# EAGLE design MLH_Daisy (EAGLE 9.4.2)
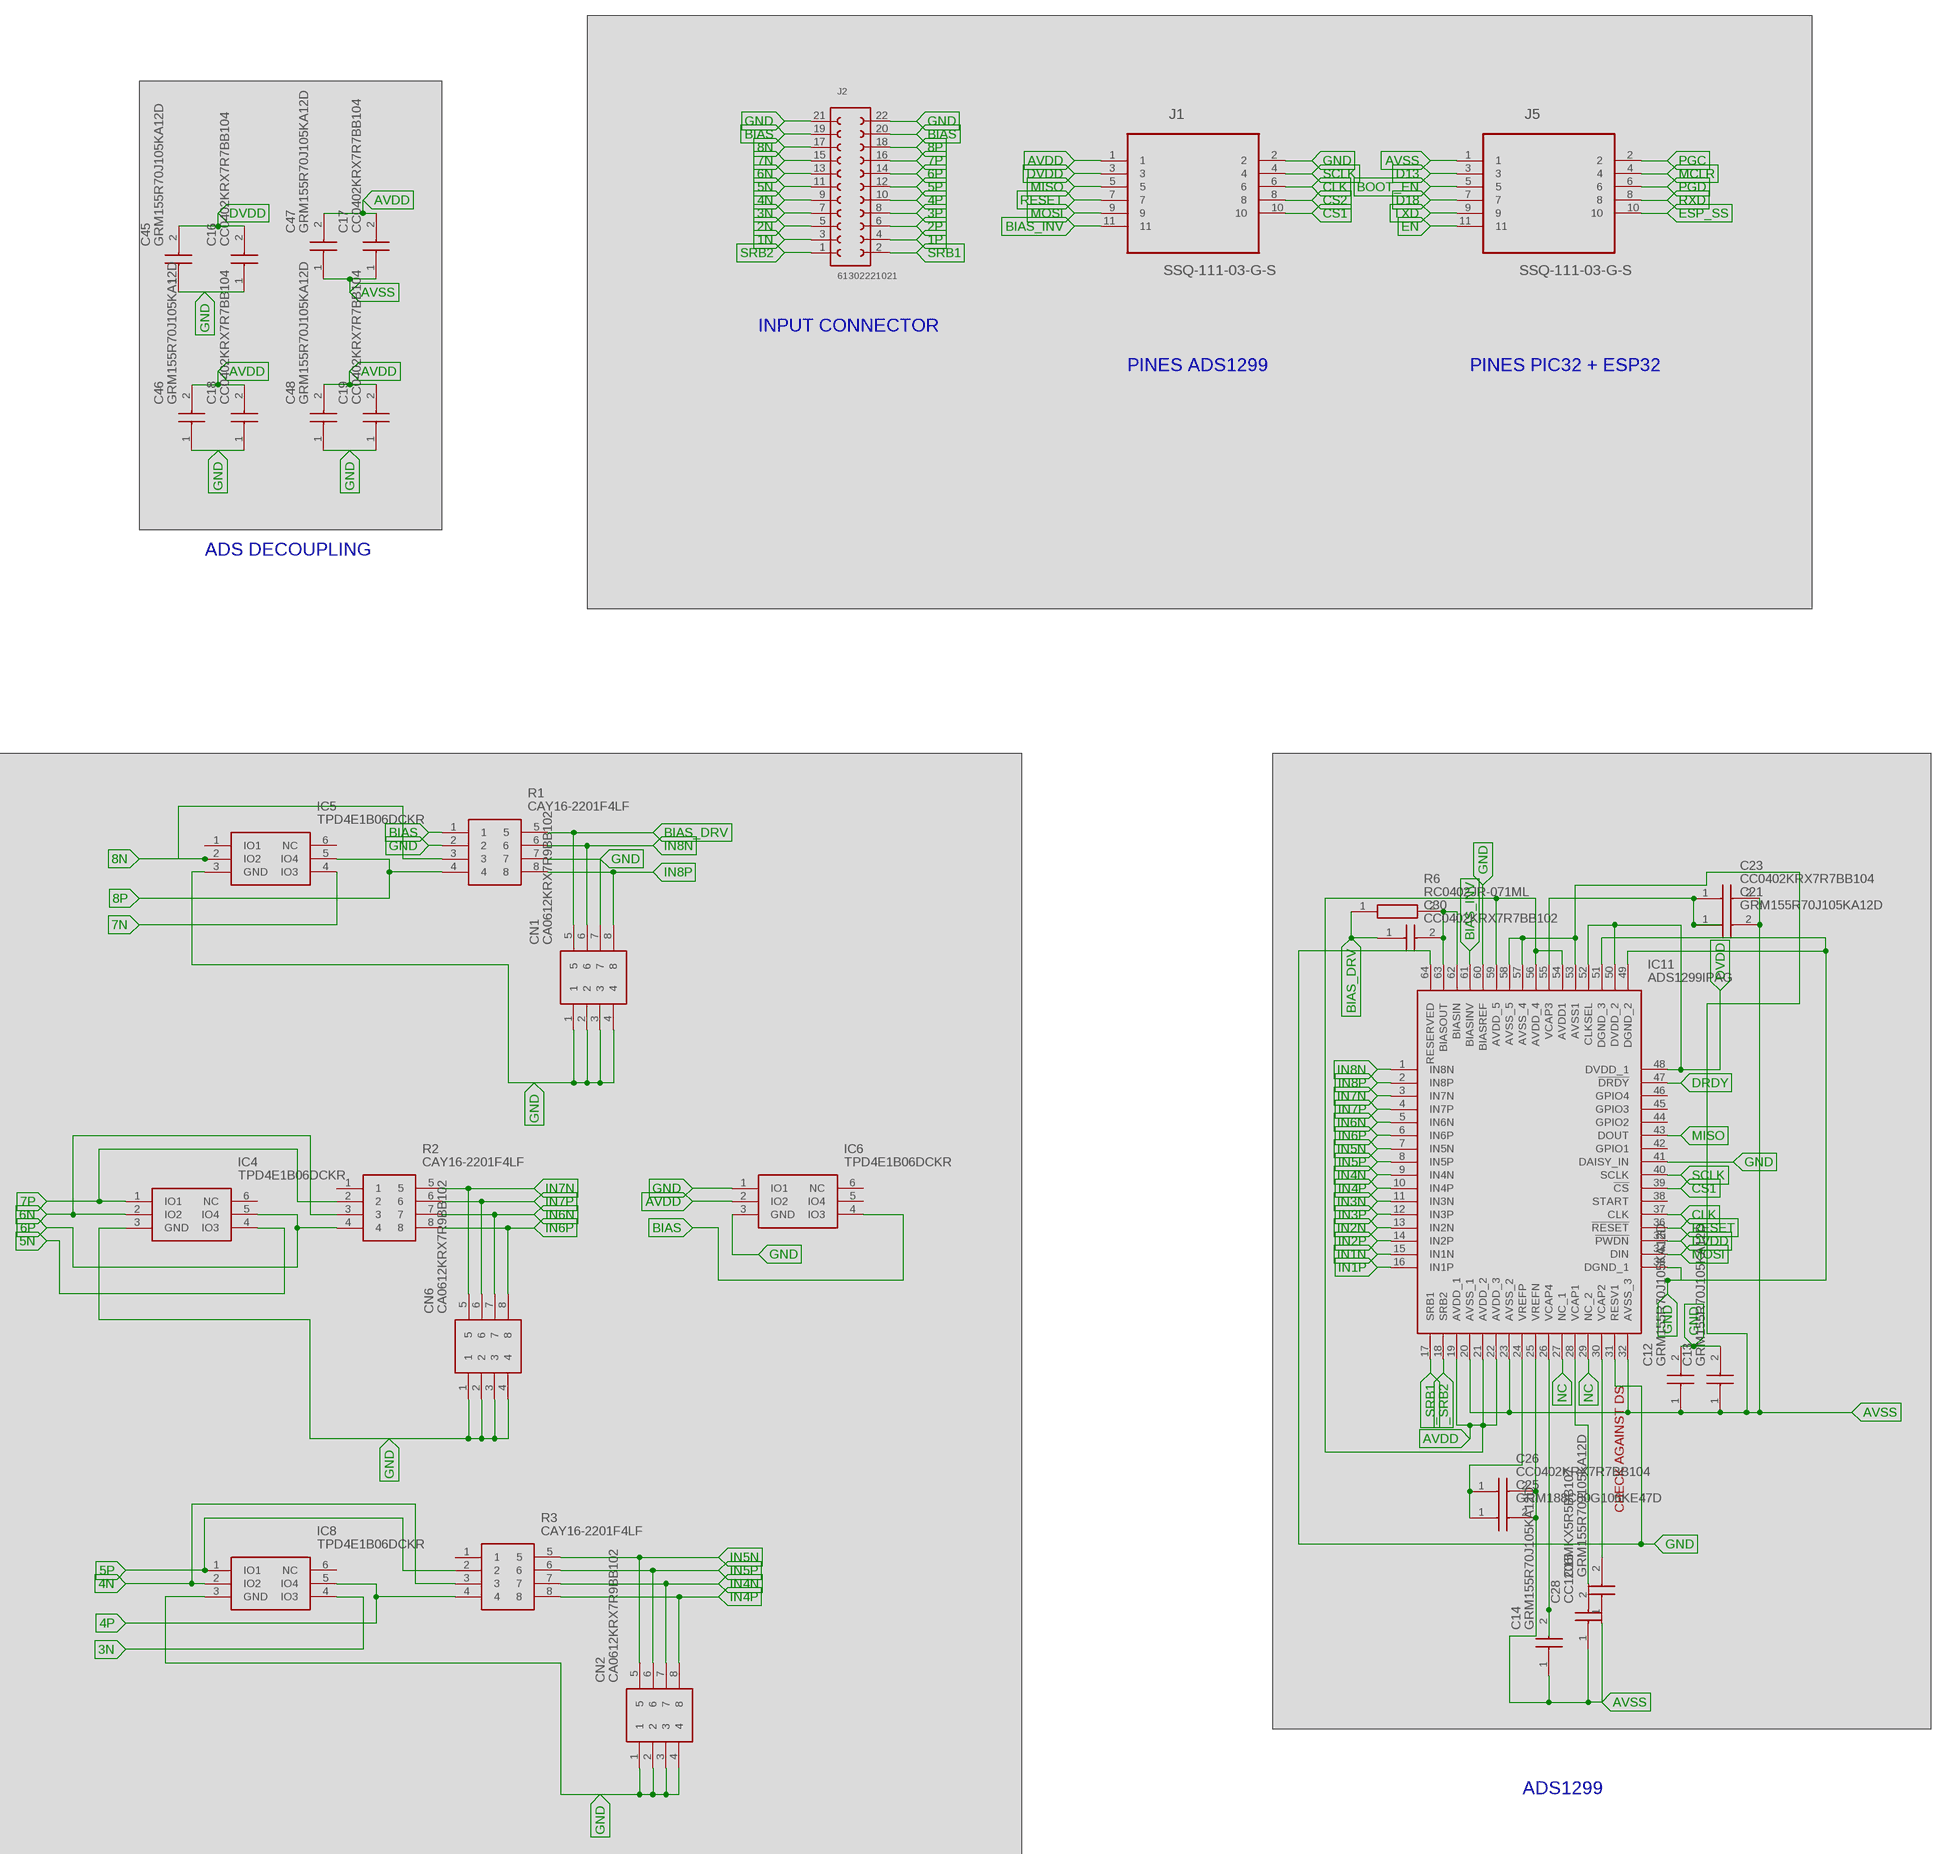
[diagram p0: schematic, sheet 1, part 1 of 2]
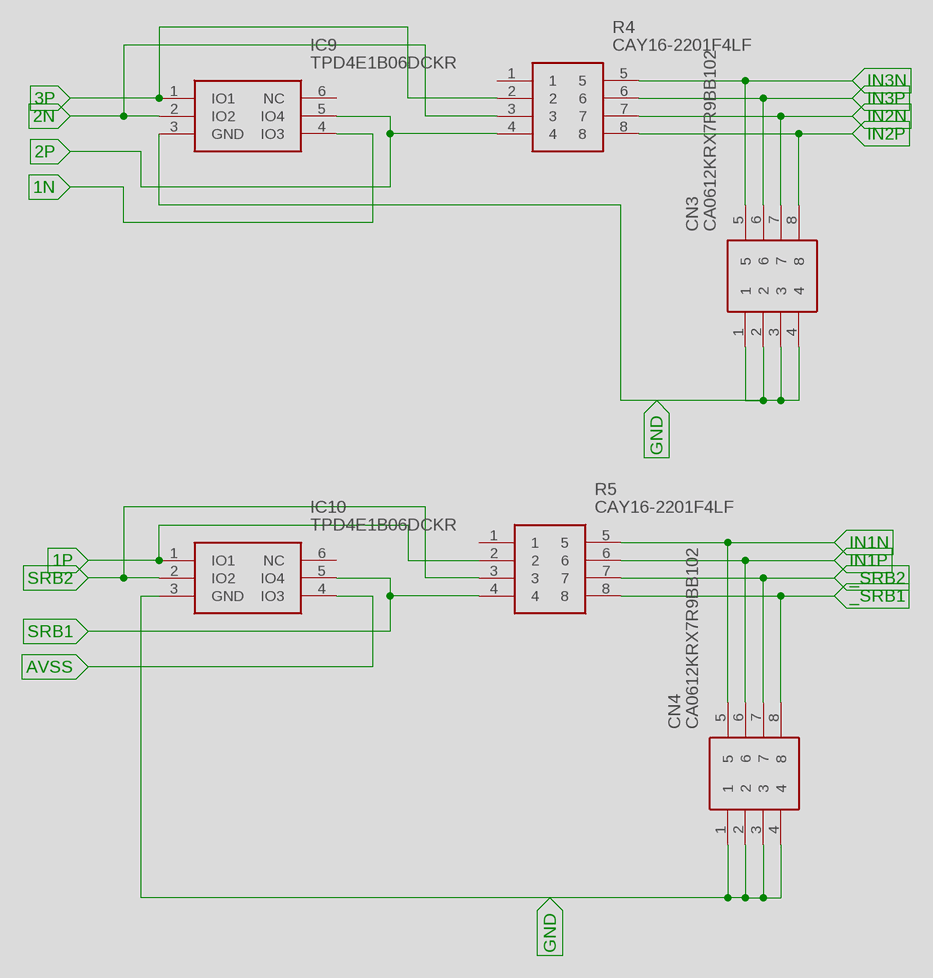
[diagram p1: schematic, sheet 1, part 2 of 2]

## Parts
C12  GRM155R70J105KA12D  [CAPC1005X55N]
C13  GRM155R70J105KA12D  [CAPC1005X55N]
C14  GRM155R70J105KA12D  [CAPC1005X55N]
C15  GRM155R70J105KA12D  [CAPC1005X55N]
C16  CC0402KRX7R7BB104  [CAPC1005X55N]
C17  CC0402KRX7R7BB104  [CAPC1005X55N]
C18  CC0402KRX7R7BB104  [CAPC1005X55N]
C19  CC0402KRX7R7BB104  [CAPC1005X55N]
C21  GRM155R70J105KA12D  [CAPC1005X55N]
C23  CC0402KRX7R7BB104  [CAPC1005X55N]
C25  GRM188C80G106KE47D  [CAPC1608X90N]
C26  CC0402KRX7R7BB104  [CAPC1005X55N]
C28  CC1206MKX5R5BB107  [CAPC3216X125N]
C30  CC0402KRX7R7BB102  [CAPC1005X55N]
C45  GRM155R70J105KA12D  [CAPC1005X55N]
C46  GRM155R70J105KA12D  [CAPC1005X55N]
C47  GRM155R70J105KA12D  [CAPC1005X55N]
C48  GRM155R70J105KA12D  [CAPC1005X55N]
CN1  CA0612KRX7R9BB102  [CA0612KRX7R9BB102]
CN2  CA0612KRX7R9BB102  [CA0612KRX7R9BB102]
CN3  CA0612KRX7R9BB102  [CA0612KRX7R9BB102]
CN4  CA0612KRX7R9BB102  [CA0612KRX7R9BB102]
CN6  CA0612KRX7R9BB102  [CA0612KRX7R9BB102]
IC4  TPD4E1B06DCKR  [SOT65P210X110-6N]
IC5  TPD4E1B06DCKR  [SOT65P210X110-6N]
IC6  TPD4E1B06DCKR  [SOT65P210X110-6N]
IC8  TPD4E1B06DCKR  [SOT65P210X110-6N]
IC9  TPD4E1B06DCKR  [SOT65P210X110-6N]
IC10  TPD4E1B06DCKR  [SOT65P210X110-6N]
IC11  ADS1299IPAG  [QFP50P1200X1200X120-64N]
J1  SSQ-111-03-G-S  [SAMTEC_SSQ-111-03-G-S]
J2  61302221021  [61302221021]
J5  SSQ-111-03-G-S  [SAMTEC_SSQ-111-03-G-S]
R1  CAY16-2201F4LF  [RESCAX80P160X320X60-8N]
R2  CAY16-2201F4LF  [RESCAX80P160X320X60-8N]
R3  CAY16-2201F4LF  [RESCAX80P160X320X60-8N]
R4  CAY16-2201F4LF  [RESCAX80P160X320X60-8N]
R5  CAY16-2201F4LF  [RESCAX80P160X320X60-8N]
R6  RC0402JR-071ML  [RESC1005X40N]

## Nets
1N: IC9.4(IO3) J2.3
1P: IC10.1(IO1) J2.4 R5.2
2N: IC9.2(IO2) J2.5 R4.3
2P: IC9.5(IO4) J2.6 R4.4
3N: IC8.4(IO3) J2.7
3P: IC9.1(IO1) J2.8 R4.2
4N: IC8.2(IO2) J2.9 R3.3
4P: IC8.5(IO4) J2.10 R3.4
5N: IC4.4(IO3) J2.11
5P: IC8.1(IO1) J2.12 R3.2
6N: IC4.2(IO2) J2.13 R2.3
6P: IC4.5(IO4) J2.14 R2.4
7N: IC5.4(IO3) J2.15
7P: IC4.1(IO1) J2.16 R2.2
8N: IC5.2(IO2) J2.17 R1.3
8P: IC5.5(IO4) J2.18 R1.4
_SRB1: CN4.8 IC11.17(SRB1) R5.8
_SRB2: CN4.7 IC11.18(SRB2) R5.7
AVDD: C17.2 C18.2 C19.2 C46.2 C47.2 C48.2 IC6.2(IO2) IC11.19(AVDD_1) IC11.21(AVDD_2) IC11.22(AVDD_3) IC11.54(AVDD1) IC11.56(AVDD_4) IC11.59(AVDD_5) J1.1
AVSS: C12.1 C13.1 C14.1 C15.1 C17.1 C21.2 C23.2 C25.2 C26.2 C28.1 C47.1 IC10.4(IO3) IC11.20(AVSS_1) IC11.23(AVSS_2) IC11.25(VREFN) IC11.32(AVSS_3) IC11.53(AVSS1) IC11.57(AVSS_4) IC11.58(AVSS_5) J5.1
BIAS: IC6.4(IO3) J2.19 J2.20 R1.1
BIAS_DRV: C30.1 CN1.5 R1.5 R6.1
BIAS_INV: IC11.61(BIASINV) J1.11
BOOT_EN: J5.5
CLK: IC11.37(CLK) J1.6
CS1: IC11.39(!CS) J1.10
CS2: J1.8
D13: J5.3
D18: J5.7
DRDY: IC11.47(!DRDY)
DVDD: C16.2 C45.2 IC11.35(!PWDN) IC11.48(DVDD_1) IC11.50(DVDD_2) IC11.52(CLKSEL) J1.3
EN: J5.11
ESP_SS: J5.10
GND: C12.2 C13.2 C16.1 C18.1 C19.1 C45.1 C46.1 C48.1 CN1.1 CN1.2 CN1.3 CN1.4 CN2.1 CN2.2 CN2.3 CN2.4 CN3.1 CN3.2 CN3.3 CN3.4 CN4.1 CN4.2 CN4.3 CN4.4 CN6.1 CN6.2 CN6.3 CN6.4 IC4.3(GND) IC5.3(GND) IC6.1(IO1) IC6.3(GND) IC8.3(GND) IC9.3(GND) IC10.3(GND) IC11.31(RESV1) IC11.33(DGND_1) IC11.41(DAISY_IN) IC11.49(DGND_2) IC11.51(DGND_3) IC11.60(BIASREF) IC11.64(RESERVED) J1.2 J2.21 J2.22 R1.2
IN1N: CN4.5 IC11.15(IN1N) R5.5
IN1P: CN4.6 IC11.16(IN1P) R5.6
IN2N: CN3.7 IC11.13(IN2N) R4.7
IN2P: CN3.8 IC11.14(IN2P) R4.8
IN3N: CN3.5 IC11.11(IN3N) R4.5
IN3P: CN3.6 IC11.12(IN3P) R4.6
IN4N: CN2.7 IC11.9(IN4N) R3.7
IN4P: CN2.8 IC11.10(IN4P) R3.8
IN5N: CN2.5 IC11.7(IN5N) R3.5
IN5P: CN2.6 IC11.8(IN5P) R3.6
IN6N: CN6.7 IC11.5(IN6N) R2.7
IN6P: CN6.8 IC11.6(IN6P) R2.8
IN7N: CN6.5 IC11.3(IN7N) R2.5
IN7P: CN6.6 IC11.4(IN7P) R2.6
IN8N: CN1.6 IC11.1(IN8N) R1.6
IN8P: CN1.8 IC11.2(IN8P) R1.8
MCLR: J5.4
MISO: IC11.43(DOUT) J1.5
MOSI: IC11.34(DIN) J1.9
N$12: CN1.7 R1.7
N$36: C21.1 C23.1 IC11.55(VCAP3)
N$39: C25.1 C26.1 IC11.24(VREFP)
N$42: C28.2 IC11.28(VCAP1)
N$43: C15.2 IC11.30(VCAP2)
N$57: C30.2 IC11.62(BIASIN) IC11.63(BIASOUT) R6.2
N$97: C14.2 IC11.26(VCAP4)
NC: IC11.27(NC_1) IC11.29(NC_2)
PGC: J5.2
PGD: J5.6
RESET: IC11.36(!RESET) J1.7
RXD: J5.8
SCLK: IC11.40(SCLK) J1.4
SRB1: IC10.5(IO4) J2.2 R5.4
SRB2: IC10.2(IO2) J2.1 R5.3
TXD: J5.9
Unconnected: IC4.6(NC) IC5.1(IO1) IC5.6(NC) IC6.5(IO4) IC6.6(NC) IC8.6(NC) IC9.6(NC) IC10.6(NC) IC11.38(START) IC11.42(GPIO1) IC11.44(GPIO2) IC11.45(GPIO3) IC11.46(GPIO4) R2.1 R3.1 R4.1 R5.1

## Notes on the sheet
- INPUT CONNECTOR
- PINES ADS1299 | PINES PIC32 + ESP32
- ADS DECOUPLING
- CHECK AGAINST DS
- ADS1299

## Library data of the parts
C12-C15 C21 C45-C48 = Cyton:GRM155R70J105KA12D: Multilayer Ceramic Capacitors MLCC - SMD/SMT 0402 1.0uF 6.3volts *Derate Voltage/Temp; DESCRIPTION: Multilayer Ceramic Capacitors MLCC - SMD/SMT 0402 1.0uF 6.3volts *Derate Voltage/Temp; HEIGHT: 0.55mm; MANUFACTURER_NAME: Murata Electronics; MANUFACTURER_PART_NUMBER: GRM155R70J105KA12D; RS_PART_NUMBER: 1138711P; RS_PRICE-STOCK: http://uk.rs-online.com/web/p/products/1138711P
C16-C19 C23 C26 = Cyton:CC0402KRX7R7BB104: Cap 100nF 16V 0402 SMD 10% X7R Phycomp 100nF Multilayer Ceramic Capacitor (MLCC) 16 V dc +/-10% X7R dielectric Standard max op. temp. +125C; DESCRIPTION: Cap 100nF 16V 0402 SMD 10% X7R Phycomp 100nF Multilayer Ceramic Capacitor (MLCC) 16 V dc +/-10% X7R dielectric Standard max op. temp. +125C; HEIGHT: 0.55mm; MANUFACTURER_NAME: YAGEO (PHYCOMP); MANUFACTURER_PART_NUMBER: CC0402KRX7R7BB104; RS_PART_NUMBER: 6169701; RS_PRICE-STOCK: https://uk.rs-online.com/web/p/products/6169701
C25 = Cyton:GRM188C80G106KE47D: Multilayer Ceramic Capacitors MLCC - SMD/SMT 0603 10uF 4volts *Derate Voltage/Temp; DESCRIPTION: Multilayer Ceramic Capacitors MLCC - SMD/SMT 0603 10uF 4volts *Derate Voltage/Temp; HEIGHT: 0.9mm; MANUFACTURER_NAME: Murata Electronics; MANUFACTURER_PART_NUMBER: GRM188C80G106KE47D; RS_PART_NUMBER: 1726485; RS_PRICE-STOCK: http://uk.rs-online.com/web/p/products/1726485
C28 = Cyton:CC1206MKX5R5BB107: Multilayer Ceramic Capacitors MLCC - SMD/SMT FACTORY NOT ACCEPTING ORDERS; DESCRIPTION: Multilayer Ceramic Capacitors MLCC - SMD/SMT FACTORY NOT ACCEPTING ORDERS; HEIGHT: 1.25mm; MANUFACTURER_NAME: YAGEO (PHYCOMP); MANUFACTURER_PART_NUMBER: CC1206MKX5R5BB107
C30 = Cyton:CC0402KRX7R7BB102: YAGEO - CC0402KRX7R7BB102 - CERAMIC CAPACITOR 1000PF, 16V, X7R, 10%, 0402, FULL REEL; DESCRIPTION: YAGEO - CC0402KRX7R7BB102 - CERAMIC CAPACITOR 1000PF, 16V, X7R, 10%, 0402, FULL REEL; HEIGHT: 0.55mm; MANUFACTURER_NAME: YAGEO (PHYCOMP); MANUFACTURER_PART_NUMBER: CC0402KRX7R7BB102
CN1-CN4 CN6 = Cyton:CA0612KRX7R9BB102: Capacitor,ceramic,multilayer,SMT,50V,1pF Source: Datasheet; DESCRIPTION: Capacitor,ceramic,multilayer,SMT,50V,1pF; HEIGHT: mm; MANUFACTURER_NAME: YAGEO (PHYCOMP); MANUFACTURER_PART_NUMBER: CA0612KRX7R9BB102; RS_PART_NUMBER: 6169789; RS_PRICE-STOCK: http://uk.rs-online.com/web/p/products/6169789
IC4-IC6 IC8-IC10 = Cyton:TPD4E1B06DCKR: Texas Instruments TPD4E1B06DCKR Quad Bi-Directional ESD Protection Array, 45W peak, 6-Pin SC-70 Source: Datasheet; DESCRIPTION: Texas Instruments TPD4E1B06DCKR Quad Bi-Directional ESD Protection Array, 45W peak, 6-Pin SC-70; HEIGHT: 1.1mm; MANUFACTURER_NAME: Texas Instruments; MANUFACTURER_PART_NUMBER: TPD4E1B06DCKR; RS_PART_NUMBER: 8255330P; RS_PRICE-STOCK: http://uk.rs-online.com/web/p/products/8255330P
IC11 = Cyton:ADS1299IPAG: Low-Noise, 8-Channel, 24-Bit Analog-to-Digital Converter for Biopotential Measurements Source: Datasheet; DESCRIPTION: Low-Noise, 8-Channel, 24-Bit Analog-to-Digital Converter for Biopotential Measurements; HEIGHT: 1.2mm; MANUFACTURER_NAME: Texas Instruments; MANUFACTURER_PART_NUMBER: ADS1299IPAG
J1 J5 = Cyton:SSQ-111-03-G-S: CONN SOCKET, 2.54MM, THT VERT, 11POS; AVAILABILITY: Unavailable; DESCRIPTION: SSQ Series .100 Tiger Buy™ Socket Strip, Square Tail; MF: Samtec; MP: SSQ-111-03-G-S; PACKAGE: None; PRICE: None
J2 = Cyton:61302221021: WR-PHD 2.54mm Angled Dual Pin Header, 22 Pins =>Code : Con_BTB_PHD_2.54_2_61302221021 Details see: http://katalog.we-online.de/en/em/613_0xx_210_21 Created 2014-05-29, Karrer Zheng 2014 (C) Würth Elektronik; AVAILABILITY: Unavailable; DESCRIPTION: WR-PHD 2.54mm Angled Dual Pin Header 22p; MF: Wurth Electronics; MP: 61302221021; PACKAGE: None; PRICE: None
R1-R5 = Cyton:CAY16-2201F4LF: Bourns CAY16 Series 2.2k +/-1% Isolated SMT Resistor Array, 4 Resistors, 0.25W total 1206 Package Convex Source: Datasheet; DESCRIPTION: Bourns CAY16 Series 2.2k +/-1% Isolated SMT Resistor Array, 4 Resistors, 0.25W total 1206 Package Convex; HEIGHT: 0.6mm; MANUFACTURER_NAME: Bourns; MANUFACTURER_PART_NUMBER: CAY16-2201F4LF; RS_PART_NUMBER: 7408773P; RS_PRICE-STOCK: http://uk.rs-online.com/web/p/products/7408773P
R6 = Cyton:RC0402JR-071ML: YAGEO RC0402 VALUE1; DESCRIPTION: YAGEO RC0402 VALUE1; HEIGHT: 0.4mm; MANUFACTURER_NAME: YAGEO (PHYCOMP); MANUFACTURER_PART_NUMBER: RC0402JR-071ML

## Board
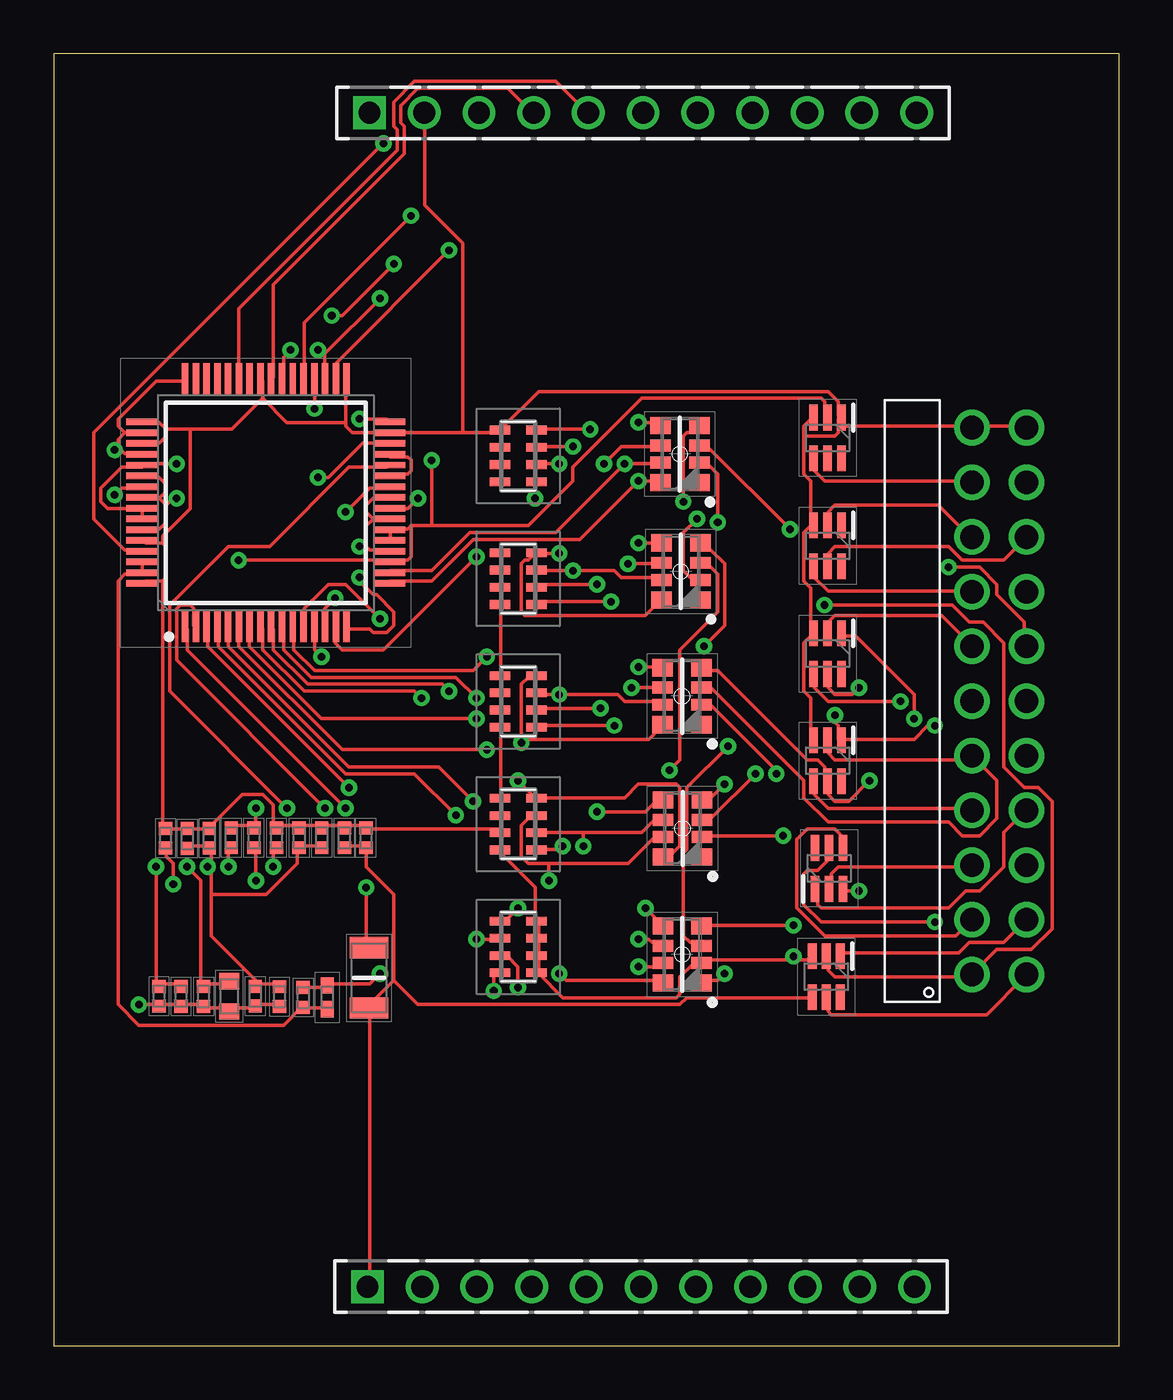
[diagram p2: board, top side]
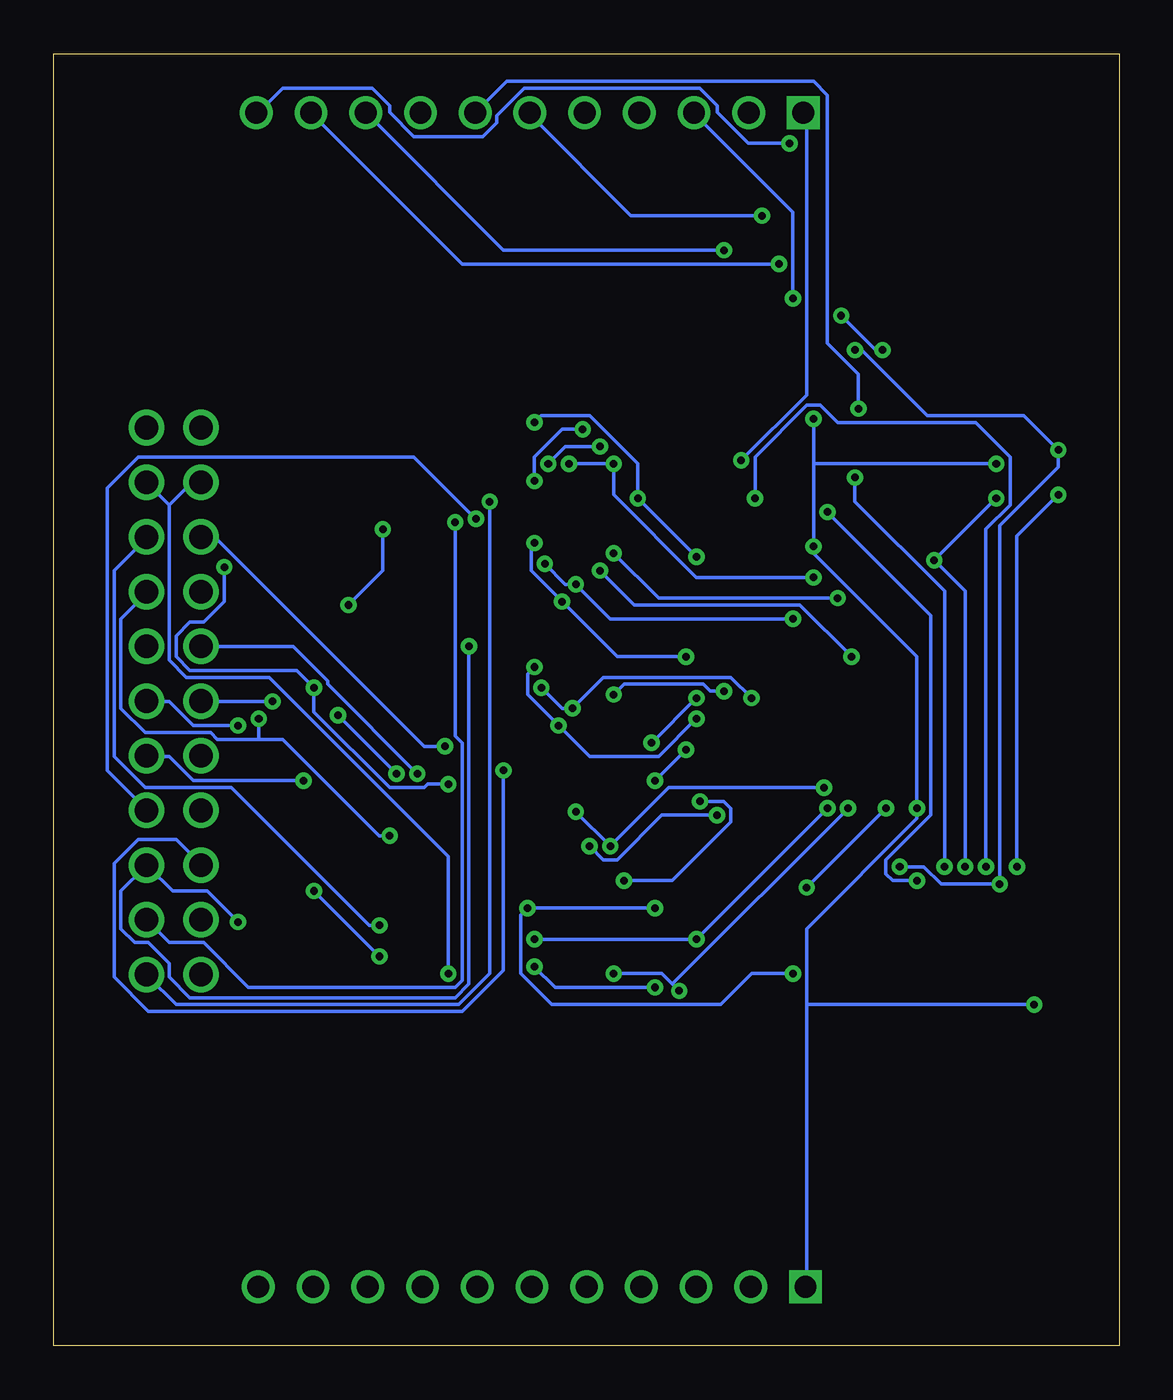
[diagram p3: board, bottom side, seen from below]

Size 49.46 x 60 mm. Coordinates in mm from the lower left corner, seen from the top.
Outline: 0,0 49.46,0 49.46,60 0,60 0,0
Copper layers (1+2*15+16): Top 0.035mm / dielectric 1.5mm / Route2 0.035mm / dielectric 0.15mm / Route15 0.035mm / dielectric 0.2mm / Bottom 0.035mm
Design rules "default *": minimum track width 6mil, minimum drill 0.35mm, track to track 6mil, track to pad 6mil, pad to pad 6mil, via to via 6mil, smd to smd 6mil, copper to edge 40mil, drill to drill 6mil, minimum pad ring 10mil, minimum via ring 8mil, stop-mask expansion 4mil, vias tented up to drill 0mil, thermal gap 10mil

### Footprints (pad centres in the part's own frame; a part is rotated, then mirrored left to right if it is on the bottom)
CAPC1005X55N = smd 0.6 x 0.62: 1 -0.46,0; 2 0.46,0
CAPC1608X90N = smd 0.75 x 0.94: 1 -0.7,0; 2 0.7,0
CAPC3216X125N = smd 0.99 x 1.78: 1 -1.4,0; 2 1.4,0
CA0612KRX7R9BB102 = smd 0.95 x 0.4: 1 -0.85,1.2; 2 -0.85,0.4; 3 -0.85,-0.4; 4 -0.85,-1.2; 5 0.85,-1.2; 6 0.85,-0.4; 7 0.85,0.4; 8 0.85,1.2
SOT65P210X110-6N = smd 1.2 x 0.4: 1 -0.95,0.65; 2 -0.95,0; 3 -0.95,-0.65; 4 0.95,-0.65; 5 0.95,0; 6 0.95,0.65
QFP50P1200X1200X120-64N = smd 1.475 x 0.3: 1 -5.738,3.75; 2 -5.738,3.25; 3 -5.738,2.75; 4 -5.738,2.25; 5 -5.738,1.75; 6 -5.738,1.25; 7 -5.738,0.75; 8 -5.738,0.25; 9 -5.738,-0.25; 10 -5.738,-0.75; 11 -5.738,-1.25; 12 -5.738,-1.75; 13 -5.738,-2.25; 14 -5.738,-2.75; 15 -5.738,-3.25; 16 -5.738,-3.75; 33 5.738,-3.75; 34 5.738,-3.25; 35 5.738,-2.75; 36 5.738,-2.25; 37 5.738,-1.75; 38 5.738,-1.25; 39 5.738,-0.75; 40 5.738,-0.25; 41 5.738,0.25; 42 5.738,0.75; 43 5.738,1.25; 44 5.738,1.75; 45 5.738,2.25; 46 5.738,2.75; 47 5.738,3.25; 48 5.738,3.75 | smd 0.3 x 1.475: 17 -3.75,-5.738; 18 -3.25,-5.738; 19 -2.75,-5.738; 20 -2.25,-5.738; 21 -1.75,-5.738; 22 -1.25,-5.738; 23 -0.75,-5.738; 24 -0.25,-5.738; 25 0.25,-5.738; 26 0.75,-5.738; 27 1.25,-5.738; 28 1.75,-5.738; 29 2.25,-5.738; 30 2.75,-5.738; 31 3.25,-5.738; 32 3.75,-5.738; 49 3.75,5.738; 50 3.25,5.738; 51 2.75,5.738; 52 2.25,5.738; 53 1.75,5.738; 54 1.25,5.738; 55 0.75,5.738; 56 0.25,5.738; 57 -0.25,5.738; 58 -0.75,5.738; 59 -1.25,5.738; 60 -1.75,5.738; 61 -2.25,5.738; 62 -2.75,5.738; 63 -3.25,5.738; 64 -3.75,5.738
SAMTEC_SSQ-111-03-G-S = drill 1.016 square: 1 -25.4,0 | drill 1.016: 2 -22.86,0; 3 -20.32,0; 4 -17.78,0; 5 -15.24,0; 6 -12.7,0; 7 -10.16,0; 8 -7.62,0; 9 -5.08,0; 10 -2.54,0; 11 0,0
61302221021 = drill 1.1: 1 12.7,-1.27; 2 12.7,1.27; 3 10.16,-1.27; 4 10.16,1.27; 5 7.62,-1.27; 6 7.62,1.27; 7 5.08,-1.27; 8 5.08,1.27; 9 2.54,-1.27; 10 2.54,1.27; 11 0,-1.27; 12 0,1.27; 13 -2.54,-1.27; 14 -2.54,1.27; 15 -5.08,-1.27; 16 -5.08,1.27; 17 -7.62,-1.27; 18 -7.62,1.27; 19 -10.16,-1.27; 20 -10.16,1.27; 21 -12.7,-1.27; 22 -12.7,1.27
RESCAX80P160X320X60-8N = smd 0.95 x 0.8: 1 -0.9,1.325; 4 -0.9,-1.325; 5 0.9,-1.325; 8 0.9,1.325 | smd 0.95 x 0.55: 2 -0.9,0.4; 3 -0.9,-0.4; 6 0.9,-0.4; 7 0.9,0.4
RESC1005X40N = smd 0.75 x 0.6: 1 -0.55,0; 2 0.55,0

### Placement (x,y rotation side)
C12  13.49,23.59 90 top
C13  14.49,23.59 90 top
C14  9.29,23.59 270 top
C15  8.24,23.59 270 top
C16  5.18,23.57 270 top
C17  9.35,16.23 90 top
C18  6.19,23.56 270 top
C19  7.22,23.57 270 top
C21  4.88,16.23 270 top
C23  5.91,16.23 270 top
C25  8.14,16.23 270 top
C26  6.95,16.22 270 top
C28  14.63,17.09 90 top
C30  11.57,16.17 270 top
C45  10.34,23.59 270 top
C46  11.39,23.59 270 top
C47  10.47,16.21 90 top
C48  12.44,23.59 270 top
CN1  21.56,18.52 180 top
CN2  21.56,29.92 0 top
CN3  21.56,35.62 0 top
CN4  21.56,41.32 0 top
CN6  21.56,24.22 0 top
IC4  35.92,32.14 270 top
IC5  35.92,37.15 270 top
IC6  35.92,42.16 270 top
IC8  35.92,27.17 270 top
IC9  35.99,22.17 90 top
IC10  35.86,17.14 270 top
IC11  9.84,39.15 90 top
J1  40.06,57.26 0 top
J2  43.89,29.94 270 top
J5  39.96,2.74 0 top
R1  29.17,18.17 180 top
R2  29.19,24.02 180 top
R3  29.17,30.16 180 top
R4  29.11,35.96 180 top
R5  29.07,41.41 180 top
R6  12.69,16.18 270 top

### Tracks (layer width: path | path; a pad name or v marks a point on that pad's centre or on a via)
1N
  Top 0.152: IC9.4 36.58,23.2 36.58,23.68 36.26,24 34.98,24 34.5,23.52 34.5,20.32 35.78,19.04 41.86,19.04 42.5,19.68 J2.3
1P  (via drill 0.35)
  Top 0.152: v30.82,38.24 30.82,40.48 30.34,40.96 30.02,40.96 R5.2 | IC10.1 36.58,18.24 42.02,18.24 42.5,18.72 44.1,18.72 45.06,19.68 J2.4
  Bottom 0.152: v30.82,38.24 30.82,28.32 30.5,28 30.5,16.96 30.82,16.64 40.42,16.64 42.5,18.72 44.1,18.72 45.06,19.68 J2.4
2N  (via drill 0.35)
  Top 0.152: v28.58,26.72 29.06,27.2 29.06,32.32 30.82,34.08 30.82,35.84 30.34,36.32 30.02,36.32 R4.3 | IC9.2 36.1,21.28 36.1,21.92 36.42,22.24 42.5,22.24 J2.5
  Bottom 0.152: v28.58,26.72 28.58,17.44 30.5,15.52 45.06,15.52 46.66,17.12 46.66,22.4 45.54,23.52 43.78,23.52 42.66,22.4 J2.5
2P  (via drill 0.35)
  Top 0.152: v30.18,32.48 31.14,33.44 31.14,36.32 30.5,36.96 30.34,36.96 R4.4 | v40.9,19.68 35.62,19.68 34.82,20.48 34.82,21.92 34.98,22.08 35.46,22.08 35.94,22.56 35.94,23.04 IC9.5
  Bottom 0.152: v30.18,32.48 30.18,16.8 30.82,16.16 43.14,16.16 44.1,17.12 44.1,17.76 45.06,18.72 45.7,18.72 46.34,19.36 46.34,21.12 45.22,22.24 J2.6 45.06,22.24 43.94,21.12 42.34,21.12 v40.9,19.68
3N
  Top 0.152: IC8.4 35.3,26.08 35.3,25.6 35.94,24.96 42.5,24.96 J2.7
3P  (via drill 0.35)
  Top 0.152: v29.86,38.4 29.22,37.76 29.22,36 29.54,35.68 29.86,35.68 R4.2 | IC9.1 35.46,21.12 35.46,20.48 35.62,20.32 41.54,20.32 42.34,21.12 42.98,21.12 44.1,22.24 44.1,23.84 45.06,24.8 J2.8
  Bottom 0.152: v29.86,38.4 32.74,41.28 45.54,41.28 46.98,39.84 46.98,26.72 45.22,24.96 J2.8
4N
  Top 0.152: R3.3 30.18,30.56 30.5,30.56 34.82,26.24 34.82,25.44 35.94,24.32 41.54,24.32 42.18,23.68 42.98,23.68 43.78,24.48 43.78,26.24 42.66,27.36 J2.9 42.5,27.36 42.34,27.2 36.26,27.2 35.94,27.52 35.94,28 IC8.2
4P  (via drill 0.35)
  Top 0.152: R3.4 30.18,31.36 30.82,31.36 34.98,27.2 35.46,27.2 35.78,26.88 35.78,26.24 IC8.5 35.94,26.08 35.94,25.6 36.26,25.28 36.9,25.28 v37.86,26.24
  Bottom 0.152: v37.86,26.24 42.98,26.24 44.1,27.36 45.06,27.36 J2.10
5N  (via drill 0.35)
  Top 0.152: v39.3,29.92 35.94,29.92 35.3,30.56 35.3,31.04 IC4.4
  Bottom 0.152: v39.3,29.92 42.5,29.92 J2.11
5P  (via drill 0.35)
  Top 0.152: v33.54,26.56 33.54,26.72 30.5,29.76 30.18,29.76 R3.2 | v36.26,29.28 36.26,28.96 36.42,28.8 36.42,28.16 IC8.1 36.58,28.16 39.94,28.16 40.58,28.8 v40.9,28.8
  Bottom 0.152: v36.26,29.28 v33.54,26.56 | v40.9,28.8 42.98,28.8 44.1,29.92 45.06,29.92 J2.12
6N  (via drill 0.35)
  Top 0.152: v32.58,26.56 30.5,24.48 30.18,24.48 R2.3 | IC4.2 35.94,33.12 35.94,33.6 36.26,33.92 41.22,33.92 42.5,32.64 J2.13
  Bottom 0.152: v32.58,26.56 36.74,30.72 36.74,30.88 38.34,32.48 42.5,32.48 J2.13
6P  (via drill 0.35)
  Top 0.152: v31.14,26.08 30.5,25.44 30.18,25.44 R2.4 | v37.38,30.56 37.06,30.24 36.26,30.24 35.94,30.56 35.94,31.04 IC4.5 | v41.54,36.16 42.98,36.16 43.78,35.36 43.78,34.88 45.06,33.6 45.06,32.64 J2.14
  Bottom 0.152: v31.14,26.08 32.1,26.08 32.26,25.92 33.86,25.92 37.38,29.44 v37.38,30.56 38.18,31.36 43.14,31.36 43.78,32 43.78,32.96 43.14,33.6 42.5,33.6 41.54,34.56 v41.54,36.16
7N
  Top 0.152: IC5.4 35.3,36.16 35.3,35.68 35.94,35.04 42.5,35.04 J2.15
7P  (via drill 0.35)
  Top 0.152: v33.86,23.68 30.18,23.68 R2.2 | v39.94,29.12 39.94,30.24 37.22,32.96 36.58,32.96 IC4.1
  Bottom 0.152: v33.86,23.68 34.34,23.68 38.82,28.16 39.94,28.16 | 39.94,28.16 41.86,28.16 42.18,28.48 45.22,28.48 46.34,29.6 46.34,33.76 45.22,34.88 J2.16 | 39.94,28.16 v39.94,29.12
8N  (via drill 0.35)
  Top 0.152: v31.3,27.84 29.38,25.92 29.38,23.04 29.22,22.88 29.22,19.04 29.54,18.72 30.02,18.72 R1.3 | IC5.2 35.94,38.24 35.94,38.72 36.26,39.04 41.06,39.04 42.5,37.6 J2.17
  Bottom 0.152: v31.3,27.84 32.26,27.84 41.86,37.44 42.5,37.44 J2.17
8P  (via drill 0.35)
  Top 0.152: v34.34,19.52 30.18,19.52 R1.4 | IC5.5 35.94,36.32 35.94,36.8 36.26,37.12 41.54,37.12 42.18,36.48 44.1,36.48 45.06,37.44 J2.18
  Bottom 0.152: v34.34,19.52 34.82,19.52 41.22,25.92 45.22,25.92 46.66,27.36 46.66,36 45.22,37.44 J2.18
_SRB1  (via drill 0.35)
  Top 0.152: v24.9,42.56 22.5,42.56 CN4.8 | R5.8 28.1,40.16 v27.14,40.16 24.42,37.44 19.46,37.44 17.54,35.52 15.62,35.52 IC11.17
  Bottom 0.152: v24.9,42.56 25.86,42.56 27.14,41.28 v27.14,40.16
_SRB2  (via drill 0.35)
  Top 0.152: v24.1,41.76 22.5,41.76 CN4.7 | R5.7 28.1,40.96 v26.5,40.96 23.3,37.76 19.3,37.76 17.54,36 15.62,36 IC11.18
  Bottom 0.152: v24.1,41.76 25.7,41.76 v26.5,40.96
AVDD  (via drill 0.35)
  Top 0.152: C48.2 12.42,23.2 11.46,23.2 C46.2 11.3,23.04 11.3,22.4 9.86,20.96 7.3,20.96 | C18.2 6.34,23.2 7.14,23.2 C19.2 7.3,23.04 7.3,22.24 | 9.54,16.8 10.34,16.8 C47.2 | 9.54,16.8 9.38,16.8 C17.2 9.54,16.8 | 7.3,20.96 7.3,19.04 9.54,16.8 | 7.3,20.96 7.3,22.24 | 5.22,39.04 5.22,38.24 4.9,37.92 4.26,37.92 IC11.59 | 4.9,39.36 5.22,39.04 | 4.9,39.36 4.26,39.36 IC11.56 | 4.9,39.36 5.22,39.68 5.22,40 4.9,40.32 4.26,40.32 IC11.54 | 16.58,38.08 17.54,38.08 | 17.54,38.08 22.02,38.08 24.1,40.16 24.1,40.8 27.3,44 35.62,44 35.78,43.84 35.78,43.2 IC6.2 | 16.58,38.08 16.42,37.92 15.62,37.92 IC11.22 15.62,37.76 15.62,37.44 IC11.21 | 16.58,38.08 16.58,36.64 16.42,36.48 15.62,36.48 IC11.19 15.46,36.48 v8.58,36.48 | 5.22,39.04 5.54,39.36 v5.7,39.36 | 17.54,38.08 v17.54,41.12 | v7.14,22.24 7.3,22.24
  Bottom 0.152: v5.7,39.36 v8.58,36.48 7.14,35.04 v7.14,22.24 | v17.54,41.12 14.5,44.16 14.5,57.12 J1.1
AVSS  (via drill 0.35)
  Top 0.152: C12.1 13.54,23.2 14.34,23.2 C13.1 14.5,23.04 14.5,22.24 15.78,20.96 15.78,16.96 | 15.78,16.96 14.66,15.84 C28.1 14.66,15.68 14.66,2.88 J5.1 | 15.78,16.96 16.9,15.84 29.06,15.84 29.38,16.16 35.14,16.16 IC10.4 | C47.1 10.34,15.84 9.38,15.84 C17.1 9.22,15.68 8.26,15.68 C25.2 8.1,15.68 6.98,15.68 C26.2 6.82,15.84 6.02,15.84 C23.2 5.86,15.84 4.9,15.84 C21.2 4.74,15.84 v3.94,15.84 | 4.1,38.88 IC11.58 | 4.1,38.88 2.5,38.88 2.18,39.2 2.18,39.84 3.14,40.8 4.1,40.8 IC11.53 4.26,40.96 v5.7,40.96 | 4.1,38.88 IC11.57 | 14.5,37.12 14.66,36.96 15.46,36.96 IC11.20 | 14.5,37.12 14.5,38.08 14.82,38.4 | 14.82,38.4 15.46,38.4 IC11.23 | 14.82,38.4 14.5,38.72 14.5,39.04 14.82,39.36 15.46,39.36 IC11.25 | C15.1 8.26,24.16 9.22,24.16 C14.1 9.38,24.16 v9.38,24.96 | v14.18,43.04 15.46,43.04 IC11.32 | v14.18,37.12 14.5,37.12
  Bottom 0.152: 14.5,15.84 14.5,2.88 J5.1 | 14.5,15.84 14.5,19.36 9.38,24.48 v9.38,24.96 9.38,32 14.18,36.8 v14.18,37.12 14.18,40.96 | 14.18,40.96 v14.18,43.04 | 14.18,40.96 v5.7,40.96 | 14.5,15.84 v3.94,15.84
BIAS  (via drill 0.35)
  Top 0.152: IC6.4 35.3,41.12 35.3,40.64 35.78,40.16 42.5,40.16 J2.19 | v31.14,17.28 30.82,16.96 30.18,16.96 R1.1
  Bottom 0.152: v31.14,17.28 31.14,22.72 39.46,31.04 43.3,31.04 44.1,31.84 44.1,39.04 | 44.1,39.04 45.06,40 J2.20 | 44.1,39.04 43.14,40 42.66,40 J2.19
BIAS_DRV  (via drill 0.35)
  Top 0.152: C30.1 11.62,16.64 12.58,16.64 R6.1 12.74,16.8 14.66,16.8 v15.14,17.28 | v21.54,20.32 21.06,19.84 20.74,19.84 CN1.5 | v27.46,20.32 28.26,19.52 R1.5
  Bottom 0.152: v21.54,20.32 v27.46,20.32 27.78,20 27.78,17.28 26.34,15.84 18.5,15.84 17.06,17.28 v15.14,17.28
BIAS_INV  (via drill 0.35)
  Top 0.152: v15.3,55.84 1.86,42.4 1.86,38.4 3.3,36.96 4.1,36.96 IC11.61
  Bottom 0.152: v15.3,55.84 17.22,55.84 18.66,57.28 18.66,57.6 19.46,58.4 27.62,58.4 28.9,57.12 28.9,56.8 29.54,56.16 32.74,56.16 33.86,57.28 33.86,57.6 34.66,58.4 38.82,58.4 39.94,57.28 J1.11
CLK  (via drill 0.35)
  Top 0.152: v16.58,52.48 11.62,47.52 11.62,44.96 IC11.37
  Bottom 0.152: v16.58,52.48 22.66,52.48 27.3,57.12 J1.6
CS1  (via drill 0.35)
  Top 0.152: v10.98,46.24 10.66,45.92 10.66,44.96 IC11.39 | v12.9,47.84 13.38,47.84 v15.78,50.24
  Bottom 0.152: v10.98,46.24 11.3,46.24 v12.9,47.84 | v15.78,50.24 30.5,50.24 37.38,57.12 J1.10
DVDD  (via drill 0.35)
  Top 0.152: 12.58,46.08 12.58,44.96 IC11.35 | v15.14,48.64 12.58,46.08 | v5.54,21.44 5.54,22.4 5.22,22.72 5.22,23.04 C16.2 | v10.18,22.24 10.18,23.04 C45.2 | 2.98,41.76 3.3,41.44 4.1,41.44 IC11.52 | 2.98,41.76 2.98,42.08 3.3,42.4 | 3.3,42.4 IC11.50 | 3.3,42.4 2.98,42.72 2.98,43.04 4.74,44.8 6.02,44.8 IC11.48 | 2.98,41.76 v2.82,41.6 | 12.58,46.08 12.42,46.08 v12.26,46.24
  Bottom 0.152: v15.14,48.64 15.14,52.64 19.62,57.12 J1.3 | v10.18,22.24 9.06,22.24 8.26,21.44 v5.54,21.44 5.54,38.08 2.82,40.8 v2.82,41.6 4.42,43.2 8.9,43.2 11.94,46.24 v12.26,46.24
GND  (via drill 0.35)
  Top 0.152: 34.34,17.92 34.98,17.92 35.14,18.08 IC10.3 | 34.34,17.92 30.18,17.92 R1.2 30.02,17.76 29.7,17.76 29.06,17.12 29.06,16.32 28.9,16.16 23.62,16.16 22.5,17.28 CN1.1 22.5,17.44 22.5,18.08 CN1.2 22.5,18.24 22.5,18.88 CN1.3 22.5,19.04 22.5,19.68 CN1.4 22.34,19.84 22.34,21.28 20.74,22.88 CN6.4 20.74,23.04 20.74,23.68 CN6.3 | v37.38,21.12 36.74,21.12 IC9.3 | 34.34,17.92 v34.34,18.08 | CN3.1 20.74,36.8 20.74,36.16 CN3.2 20.74,36 20.74,35.36 CN3.3 20.74,35.2 20.74,34.56 CN3.4 20.74,34.4 20.74,31.2 CN2.1 20.74,31.04 20.74,30.4 CN2.2 20.74,30.24 20.74,29.6 CN2.3 20.74,29.44 20.74,28.8 CN2.4 20.74,28.64 20.74,25.44 CN6.1 20.74,25.28 20.74,24.64 CN6.2 20.74,24.48 20.74,24 | 20.74,24 20.74,23.84 CN6.3 | 20.74,24 14.5,24 C13.2 14.34,24.16 13.54,24.16 C12.2 13.38,24.16 12.58,24.16 C48.1 12.42,24.16 11.46,24.16 C46.1 11.3,24.16 10.34,24.16 C45.1 10.18,24.16 10.18,25.12 9.7,25.6 8.74,25.6 7.3,24.16 C19.1 7.14,24 6.34,24 C18.1 6.18,24 5.22,24 C16.1 5.06,24.16 5.06,35.52 | 20.74,24 CN6.3 | J2.22 45.06,42.72 42.66,42.72 J2.21 42.5,42.72 36.42,42.72 | IC8.3 35.14,28.16 35.14,30.08 34.82,30.4 34.82,32.64 35.14,32.96 IC4.3 35.14,33.12 35.14,35.2 34.82,35.52 34.82,37.76 35.14,38.08 IC5.3 35.14,38.24 35.14,40.16 34.82,40.48 34.82,42.24 | 34.82,42.24 34.82,42.72 35.14,43.04 IC6.3 | 36.42,42.72 36.42,42.4 36.26,42.24 34.82,42.24 | 36.42,42.72 36.42,43.04 IC6.1 | 36.42,42.72 IC6.1 | 5.06,35.52 4.26,35.52 IC11.64 | 5.06,35.52 5.22,35.68 5.22,37.12 5.06,37.28 | 5.06,37.28 4.26,37.28 IC11.60 | 5.22,42.56 5.22,42.24 4.9,41.92 4.26,41.92 IC11.51 | 5.22,42.56 4.9,42.88 4.26,42.88 IC11.49
  Top 0.152: CN4.4 20.74,40.16 20.74,40.8 CN4.3 20.74,40.96 20.74,41.6 CN4.2 20.74,41.76 20.74,42.4 CN4.1 | 13.54,42.88 13.54,44.8 IC11.33 | 13.54,42.88 13.54,42.72 13.86,42.4 15.46,42.4 IC11.31 15.62,42.4 18.98,42.4 | 9.7,44 9.7,44.8 IC11.41 | 9.7,44 10.82,42.88 13.54,42.88 | 18.98,42.4 20.58,42.4 CN4.1 | 6.34,42.56 8.26,42.56 9.7,44 | 6.34,42.56 5.22,42.56 | 5.06,37.28 5.06,37.6 6.34,38.88 6.34,42.56 | 18.98,42.4 18.98,51.2 17.22,52.96 17.22,57.12 J1.2 | IC6.1 36.42,43.2 36.42,43.84 35.94,44.32 22.5,44.32 20.74,42.56 CN4.1
  Bottom 0.152: v34.34,18.08 v37.38,21.12
IN1N  (via drill 0.35)
  Top 0.152: v22.34,39.36 22.34,40 CN4.5 | v27.14,42.88 28.1,42.88 R5.5 | v19.62,36.64 15.3,32.32 13.38,32.32 13.06,32.64 13.06,33.28 IC11.15
  Bottom 0.152: v27.14,42.88 26.82,43.2 24.58,43.2 22.34,40.96 v22.34,39.36 v19.62,36.64
IN1P  (via drill 0.35)
  Top 0.152: v23.46,40.96 22.5,40.96 CN4.6 | v25.54,40.96 26.34,41.76 28.1,41.76 R5.6 | v14.18,35.68 14.18,35.52 14.82,34.88 14.98,34.88 15.78,34.08 15.78,33.44 15.46,33.12 14.82,33.12 14.66,33.28 13.7,33.28 IC11.16
  Bottom 0.152: v25.54,40.96 v23.46,40.96 23.46,39.52 19.62,35.68 v14.18,35.68
IN2N  (via drill 0.35)
  Top 0.152: CN3.7 22.5,36 v24.1,36 26.02,36 26.34,35.68 28.1,35.68 R4.7 | v12.42,32 12.1,32.32 12.1,33.28 IC11.13
  Bottom 0.152: v12.42,32 14.82,34.4 22.5,34.4 v24.1,36
IN2P  (via drill 0.35)
  Top 0.152: R4.8 28.1,34.56 27.46,33.92 21.86,33.92 21.7,34.08 21.7,36.32 21.86,36.48 22.02,36.48 22.34,36.8 CN3.8 22.5,36.8 v23.46,36.8 | v13.06,34.72 12.58,34.24 12.58,33.44 IC11.14
  Bottom 0.152: v13.06,34.72 21.38,34.72 v23.46,36.8
IN3N  (via drill 0.35)
  Top 0.152: v25.86,34.56 22.5,34.56 CN3.5 | v27.14,37.28 28.1,37.28 R4.5 | v20.1,32 19.46,31.36 12.1,31.36 11.14,32.32 11.14,33.28 IC11.11
  Bottom 0.152: v27.14,37.28 27.3,37.12 27.3,36 v25.86,34.56 23.3,32 v20.1,32
IN3P  (via drill 0.35)
  Top 0.152: v25.22,35.36 22.5,35.36 CN3.6 | v26.66,36.32 28.1,36.32 R4.6 | v15.14,33.76 13.54,35.36 12.74,35.36 11.62,34.24 11.62,33.44 IC11.12
  Bottom 0.152: v26.66,36.32 25.7,35.36 v25.22,35.36 23.62,33.76 v15.14,33.76
IN4N  (via drill 0.35)
  Top 0.152: CN2.7 22.5,30.24 v23.46,30.24 26.18,30.24 26.5,29.92 28.26,29.92 R3.7 | v18.34,30.4 18.02,30.72 11.78,30.72 10.18,32.32 10.18,33.28 IC11.9
  Bottom 0.152: v18.34,30.4 18.98,30.4 19.3,30.72 22.98,30.72 v23.46,30.24
IN4P  (via drill 0.35)
  Top 0.152: 21.86,28.16 21.7,28.32 21.7,30.72 22.02,31.04 22.34,31.04 CN2.8 | 21.86,28.16 27.62,28.16 28.26,28.8 R3.8 | v19.62,30.08 18.66,31.04 11.94,31.04 10.66,32.32 10.66,33.28 IC11.10 | 21.86,28.16 v21.7,28
  Bottom 0.152: v21.7,28 v19.62,30.08
IN5N  (via drill 0.35)
  Top 0.152: v26.02,28.8 22.5,28.8 CN2.5 | v27.14,31.52 28.26,31.52 R3.5 | v19.62,29.12 12.42,29.12 9.06,32.48 9.06,33.28 IC11.7
  Bottom 0.152: v27.14,31.52 27.46,31.2 27.46,30.24 v26.02,28.8 24.58,27.36 21.38,27.36 v19.62,29.12
IN5P  (via drill 0.35)
  Top 0.152: v25.38,29.6 22.5,29.6 CN2.6 | v26.82,30.56 R3.6 | v17.06,30.08 16.74,30.4 11.62,30.4 9.7,32.32 9.7,33.28 IC11.8
  Bottom 0.152: v26.82,30.56 25.86,29.6 v25.38,29.6 23.94,31.04 18.02,31.04 v17.06,30.08
IN6N  (via drill 0.35)
  Top 0.152: 22.98,22.4 26.66,22.4 27.78,23.52 28.26,23.52 R2.7 | 22.98,22.4 22.02,22.4 21.7,22.72 21.7,24.16 22.02,24.48 22.34,24.48 CN6.7 | v19.46,25.28 17.86,26.88 13.7,26.88 8.1,32.48 8.1,33.28 IC11.5 | 22.98,22.4 v22.98,21.6
  Bottom 0.152: v19.46,25.28 18.34,25.28 18.02,24.96 18.02,24.32 20.74,21.6 v22.98,21.6
IN6P  (via drill 0.35)
  Top 0.152: R2.8 28.42,22.56 29.06,23.2 29.06,25.92 28.9,26.08 27.14,26.08 26.5,25.44 22.5,25.44 CN6.8 22.34,25.44 v21.54,26.24 | v20.1,27.68 13.38,27.68 8.58,32.48 8.58,33.28 IC11.6
  Bottom 0.152: v21.54,26.24 v20.1,27.68
IN7N  (via drill 0.35)
  Top 0.152: v23.62,23.2 23.46,23.04 22.5,23.04 CN6.5 | v25.22,24.8 27.46,24.8 27.94,25.28 28.26,25.28 R2.5 | v13.7,25.92 7.14,32.48 7.14,33.28 IC11.3
  Bottom 0.152: v25.22,24.8 v23.62,23.2 20.9,25.92 v13.7,25.92
IN7P  (via drill 0.35)
  Top 0.152: 24.58,23.84 27.3,23.84 27.78,24.32 28.26,24.32 R2.6 | 24.58,23.84 22.5,23.84 CN6.6 | v18.66,24.64 16.74,26.56 13.54,26.56 7.62,32.48 7.62,33.28 IC11.4 | 24.58,23.84 v24.58,23.2
  Bottom 0.152: v18.66,24.64 21.22,24.64 23.3,22.56 23.94,22.56 v24.58,23.2
IN8N  (via drill 0.35)
  Top 0.152: v19.62,18.88 20.58,18.88 CN1.6 | v27.14,18.88 27.62,18.88 27.78,18.72 28.26,18.72 R1.6 | v13.54,24.96 6.18,32.32 6.18,33.28 IC11.1
  Bottom 0.152: v27.14,18.88 v19.62,18.88 v13.54,24.96
IN8P  (via drill 0.35)
  Top 0.152: v23.46,17.28 23.78,16.96 28.26,16.96 R1.8 | v20.42,16.48 20.42,17.12 20.58,17.28 CN1.8 | v12.58,24.96 5.7,31.84 5.7,34.24 5.86,34.4 6.34,34.4 6.5,34.24 6.5,33.44 IC11.2
  Bottom 0.152: v23.46,17.28 21.22,17.28 20.74,16.8 | v20.42,16.48 20.74,16.8 | 20.74,16.8 v12.58,24.96
MISO
  Top 0.152: IC11.43 8.58,44.96 8.58,48.16 15.94,55.52 15.94,56.48 15.78,56.64 15.78,57.76 16.74,58.72 23.3,58.72 24.74,57.28 J1.5
MOSI  (via drill 0.35)
  Top 0.152: v18.34,50.88 13.06,45.6 13.06,44.96 IC11.34
  Bottom 0.152: v18.34,50.88 28.58,50.88 34.82,57.12 J1.9
N$12  (via drill 0.35)
  Top 0.152: v21.54,16.64 21.54,17.6 21.06,18.08 20.74,18.08 CN1.7 | v27.14,17.6 28.1,17.6 R1.7
  Bottom 0.152: v21.54,16.64 26.18,16.64 v27.14,17.6
N$36  (via drill 0.35)
  Top 0.152: C23.1 5.86,16.8 4.9,16.8 C21.1 4.74,16.8 v4.74,22.24 | v2.82,39.52 3.14,39.84 4.1,39.84 IC11.55
  Bottom 0.152: v4.74,22.24 4.74,37.6 v2.82,39.52
N$39  (via drill 0.35)
  Top 0.152: C25.1 8.1,16.8 6.98,16.8 C26.1 6.82,16.8 6.82,21.6 v6.18,22.24 | v16.9,39.36 16.42,38.88 15.62,38.88 IC11.24
  Bottom 0.152: v6.18,22.24 6.18,37.92 5.06,39.04 5.06,41.28 6.66,42.88 13.06,42.88 13.86,43.68 14.5,43.68 16.9,41.28 v16.9,39.36
N$42  (via drill 0.35)
  Top 0.152: v10.82,24.96 5.38,30.4 5.38,34.4 8.1,37.12 10.02,37.12 13.7,40.8 15.46,40.8 IC11.28 | v14.5,21.28 14.5,18.56 C28.2
  Bottom 0.152: v14.5,21.28 v10.82,24.96
N$43  (via drill 0.35)
  Top 0.152: v8.1,22.24 8.1,23.04 C15.2 | v12.26,40.32 12.74,40.32 14.34,41.92 15.46,41.92 IC11.30
  Bottom 0.152: v8.1,22.24 8.1,35.04 12.26,39.2 v12.26,40.32
N$57
  Top 0.152: R6.2 12.58,15.68 11.62,15.68 C30.2 11.46,15.68 10.66,14.88 3.94,14.88 2.98,15.84 2.98,35.52 3.3,35.84 4.1,35.84 IC11.63 4.1,36 4.1,36.32 IC11.62
N$97  (via drill 0.35)
  Top 0.152: v9.38,21.6 9.38,23.04 C14.2 | v13.54,38.72 14.66,39.84 15.46,39.84 IC11.26
  Bottom 0.152: v9.38,21.6 10.5,21.6 10.82,21.92 10.82,22.56 8.74,24.64 8.74,33.92 v13.54,38.72
NC
  Top 0.152: IC11.27 15.62,40.48 16.42,40.48 16.58,40.64 16.58,41.12 16.42,41.28 15.62,41.28 IC11.29
RESET  (via drill 0.35)
  Top 0.152: v12.1,43.52 12.1,44.8 IC11.36
  Bottom 0.152: v12.1,43.52 12.1,45.12 13.54,46.56 13.54,58.08 14.18,58.72 28.42,58.72 29.86,57.28 J1.7
SCLK
  Top 0.152: IC11.40 10.18,44.96 10.18,49.28 16.26,55.36 16.26,56.64 16.1,56.8 16.1,57.6 16.9,58.4 21.06,58.4 22.18,57.28 J1.4
SRB1  (via drill 0.35)
  Top 0.152: v29.22,39.2 29.22,42.24 29.38,42.4 29.54,42.4 29.86,42.72 R5.4 | IC10.5 35.94,16.16 35.94,15.52 36.1,15.36 43.3,15.36 45.06,17.12 J2.2
  Bottom 0.152: v29.22,39.2 29.22,17.28 30.66,15.84 43.78,15.84 45.06,17.12 J2.2
SRB2  (via drill 0.35)
  Top 0.152: v34.18,37.92 30.34,41.76 30.02,41.76 R5.3 | v35.78,34.4 41.7,34.4 42.5,33.6 43.14,33.6 44.1,32.64 44.1,26.88 45.06,25.92 45.7,25.92 46.34,25.28 46.34,19.36 45.38,18.4 43.78,18.4 42.66,17.28 J2.1 42.5,17.12 36.26,17.12 35.94,17.44 35.94,18.08 IC10.2
  Bottom 0.152: v34.18,37.92 34.18,36 v35.78,34.4

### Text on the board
space: AVDD | GND | DVDD | SCLK | CLK | RESET | CS2 | MOSI | BIAS-INV | MISO | CS1 | Do things that no one imagines | AVSS | PGC | D13 | MCLR | BOOT-EN | PGD | D18 | RXD | TXD | ESP-SS | WIFI-RST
